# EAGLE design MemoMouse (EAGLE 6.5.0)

## Sheet 1 of 2: CPU
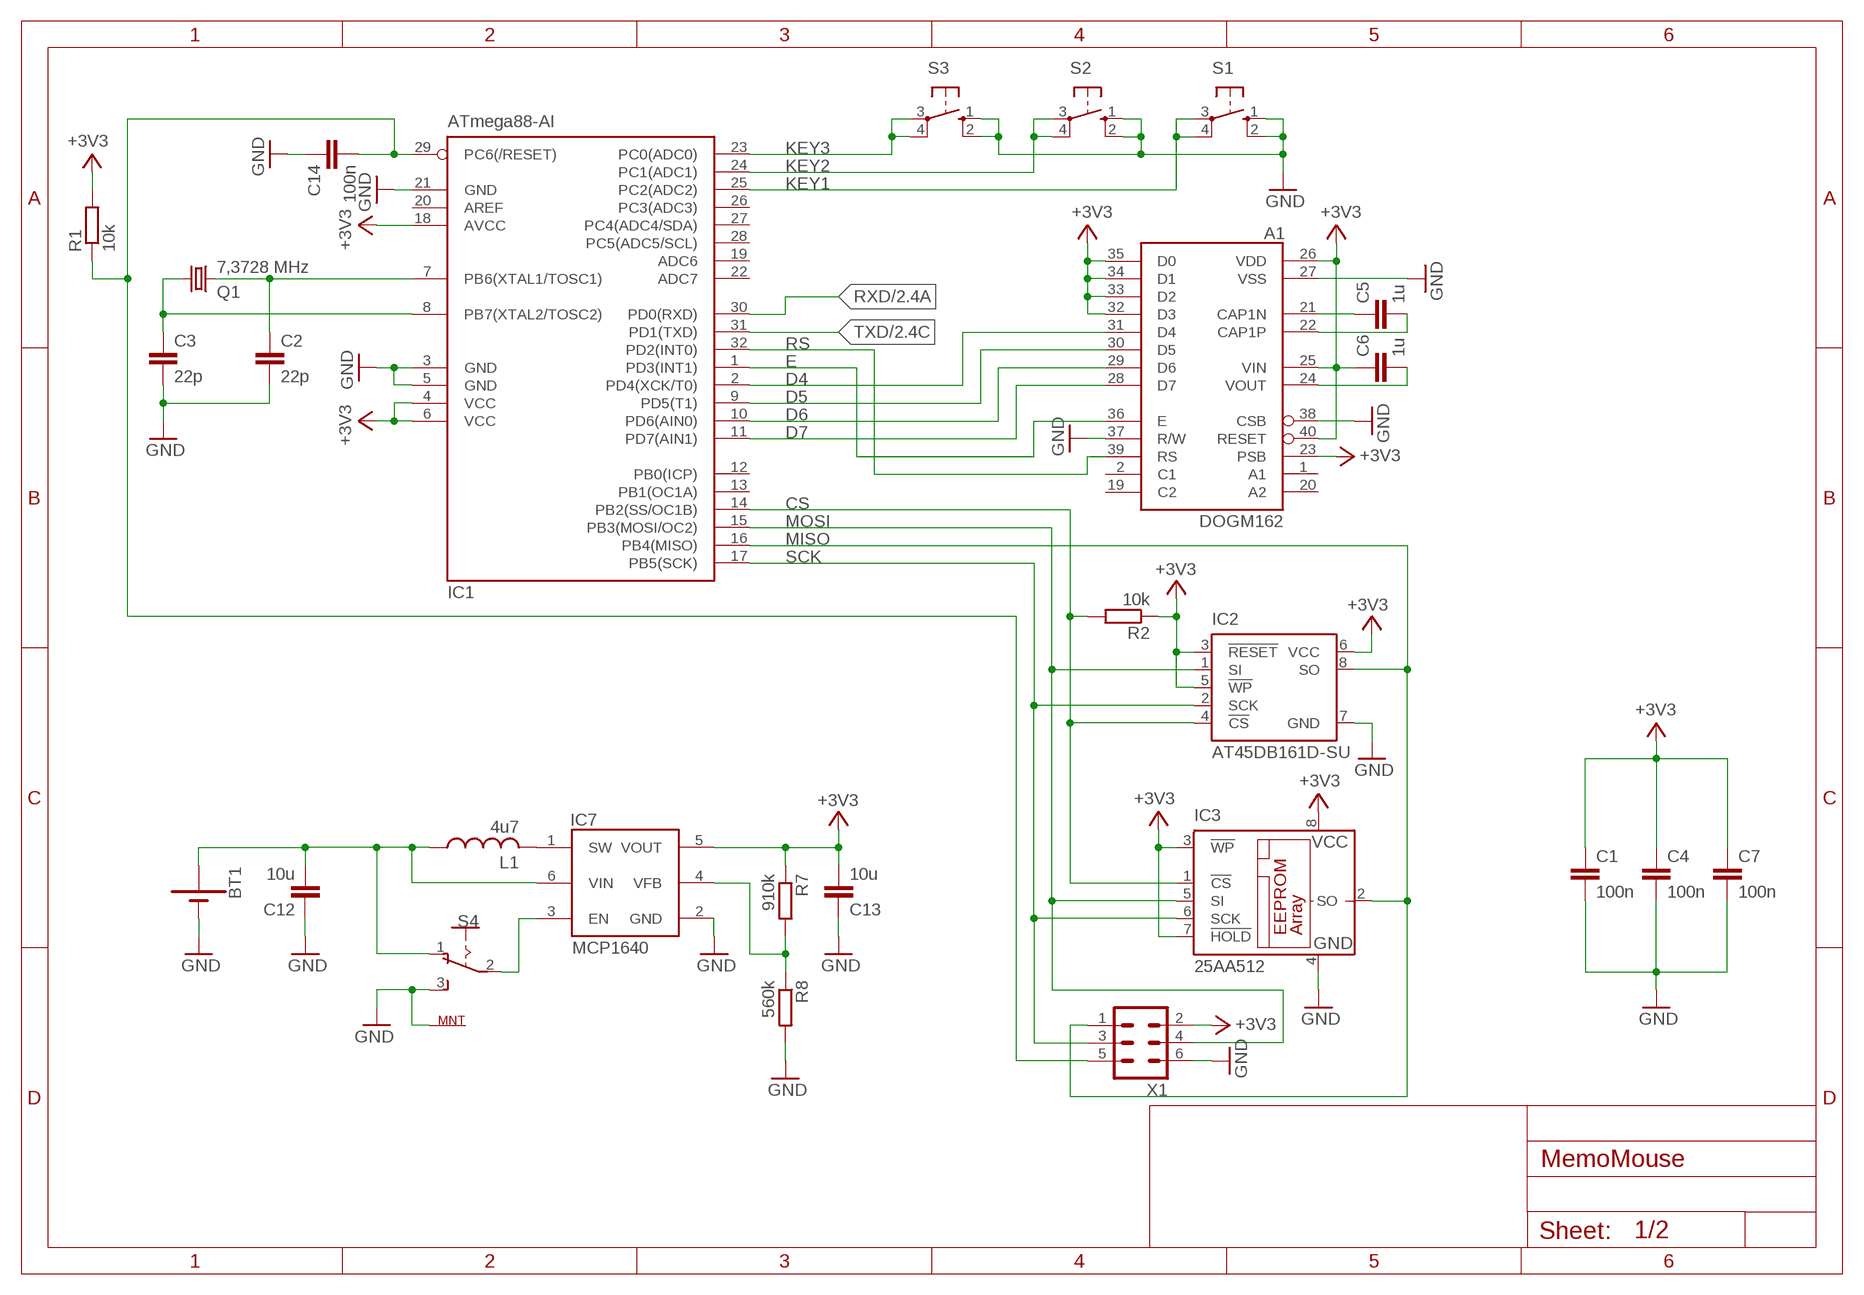
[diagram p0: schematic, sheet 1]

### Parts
A1  DOGM162  SELFMADE_DOGM  [SELFMADE_DOGM]
BT1  BATTERY-AAA_KIT  [BATTERY-AAA-KIT]
C1  100n  C-EUC0603  [C0603]
C2  22p  C-EUC0603  [C0603]
C3  22p  C-EUC0603  [C0603]
C4  100n  C-EUC0603  [C0603]
C5  1u  C-EUC0603  [C0603]
C6  1u  C-EUC0603  [C0603]
C7  100n  C-EUC0603  [C0603]
C12  10u  C-EUC0805K  [C0805K]
C13  10u  C-EUC0805K  [C0805K]
C14  100n  C-EUC0603  [C0603]
IC1  ATmega88-AI  MEGA8-AI  [TQFP32-08]
IC2  AT45DB161D-SU  [8S2]
IC3  25AA512  25AA080SN  [SO-08]
IC7  MCP1640  [SOT23-6]
L1  4u7  L-USL3225M  [L3225M]
Q1  7,3728 MHz  CRYSTALCTS406  [CTS406]
R1  10k  R-EU_R0603  [R0603]
R2  10k  R-EU_R0603  [R0603]
R7  910k  R-EU_R0603  [R0603]
R8  560k  R-EU_R0603  [R0603]
S1  10-XX  [B3F-10XX]
S2  10-XX  [B3F-10XX]
S3  10-XX  [B3F-10XX]
S4  M251SW_H  [MINI_SWITCH]
X1  MICROMATCH06  [MICROMATCH_SMD6]

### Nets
!RESET: C14.2 IC1.29(PC6(/RESET)) R1.1 X1.5
+3V3: A1.23(PSB) A1.25(VIN) A1.26(VDD) A1.32(D3) A1.33(D2) A1.34(D1) A1.35(D0) A1.40(RESET) C1.1 C4.1 C6.1 C7.1 C13.2 IC1.4(VCC) IC1.6(VCC) IC1.18(AVCC) IC2.3(!RESET) IC2.5(!WP) IC2.6(VCC) IC3.3(!WP) IC3.7(!HOLD) IC3.8(VCC) IC7.5(VOUT) R1.2 R2.1 R7.1 X1.2 ; also sheet 2
CS: IC1.14(PB2(SS/OC1B)) IC2.4(!CS) IC3.1(!CS) R2.2
D4: A1.31(D4) IC1.2(PD4(XCK/T0))
D5: A1.30(D5) IC1.9(PD5(T1))
D6: A1.29(D6) IC1.10(PD6(AIN0))
D7: A1.28(D7) IC1.11(PD7(AIN1))
E: A1.36(E) IC1.1(PD3(INT1))
GND: A1.27(VSS) A1.37(R/W) A1.38(CSB) BT1.N1(-) BT1.N2(-) C1.2 C2.2 C3.2 C4.2 C7.2 C12.1 C13.1 C14.1 IC1.3(GND) IC1.5(GND) IC1.21(GND) IC2.7(GND) IC3.4(GND) IC7.2(GND) R8.2 S1.1(S) S1.2(S1) S2.1(S) S2.2(S1) S3.1(S) S3.2(S1) S4.3(S) S4.M1(MNT) S4.M2(MNT) X1.6 ; also sheet 2
KEY1: IC1.25(PC2(ADC2)) S1.3(P) S1.4(P1)
KEY2: IC1.24(PC1(ADC1)) S2.3(P) S2.4(P1)
KEY3: IC1.23(PC0(ADC0)) S3.3(P) S3.4(P1)
MISO: IC1.16(PB4(MISO)) IC2.8(SO) IC3.2(SO) X1.1
MOSI: IC1.15(PB3(MOSI/OC2)) IC2.1(SI) IC3.5(SI) X1.4
N$8: IC7.1(SW) L1.2
N$9: A1.21(CAP1N) C5.1
N$10: A1.22(CAP1P) C5.2
N$11: A1.24(VOUT) C6.2
N$12: C2.1 IC1.7(PB6(XTAL1/TOSC1)) Q1.3
N$13: C3.1 IC1.8(PB7(XTAL2/TOSC2)) Q1.1
N$15: IC7.4(VFB) R7.2 R8.1
N$16: BT1.P1(+) BT1.P2(+) C12.2 IC7.6(VIN) L1.1 S4.1(O)
N$17: IC7.3(EN) S4.2(P)
RS: A1.39(RS) IC1.32(PD2(INT0))
RXD: IC1.30(PD0(RXD)) ; also sheet 2
SCK: IC1.17(PB5(SCK)) IC2.2(SCK) IC3.6(SCK) X1.3
TXD: IC1.31(PD1(TXD)) ; also sheet 2
Unconnected: A1.1(A1) A1.2(C1) A1.19(C2) A1.20(A2) IC1.12(PB0(ICP)) IC1.13(PB1(OC1A)) IC1.19(ADC6) IC1.20(AREF) IC1.22(ADC7) IC1.26(PC3(ADC3)) IC1.27(PC4(ADC4/SDA)) IC1.28(PC5(ADC5/SCL))

## Sheet 2 of 2: IO
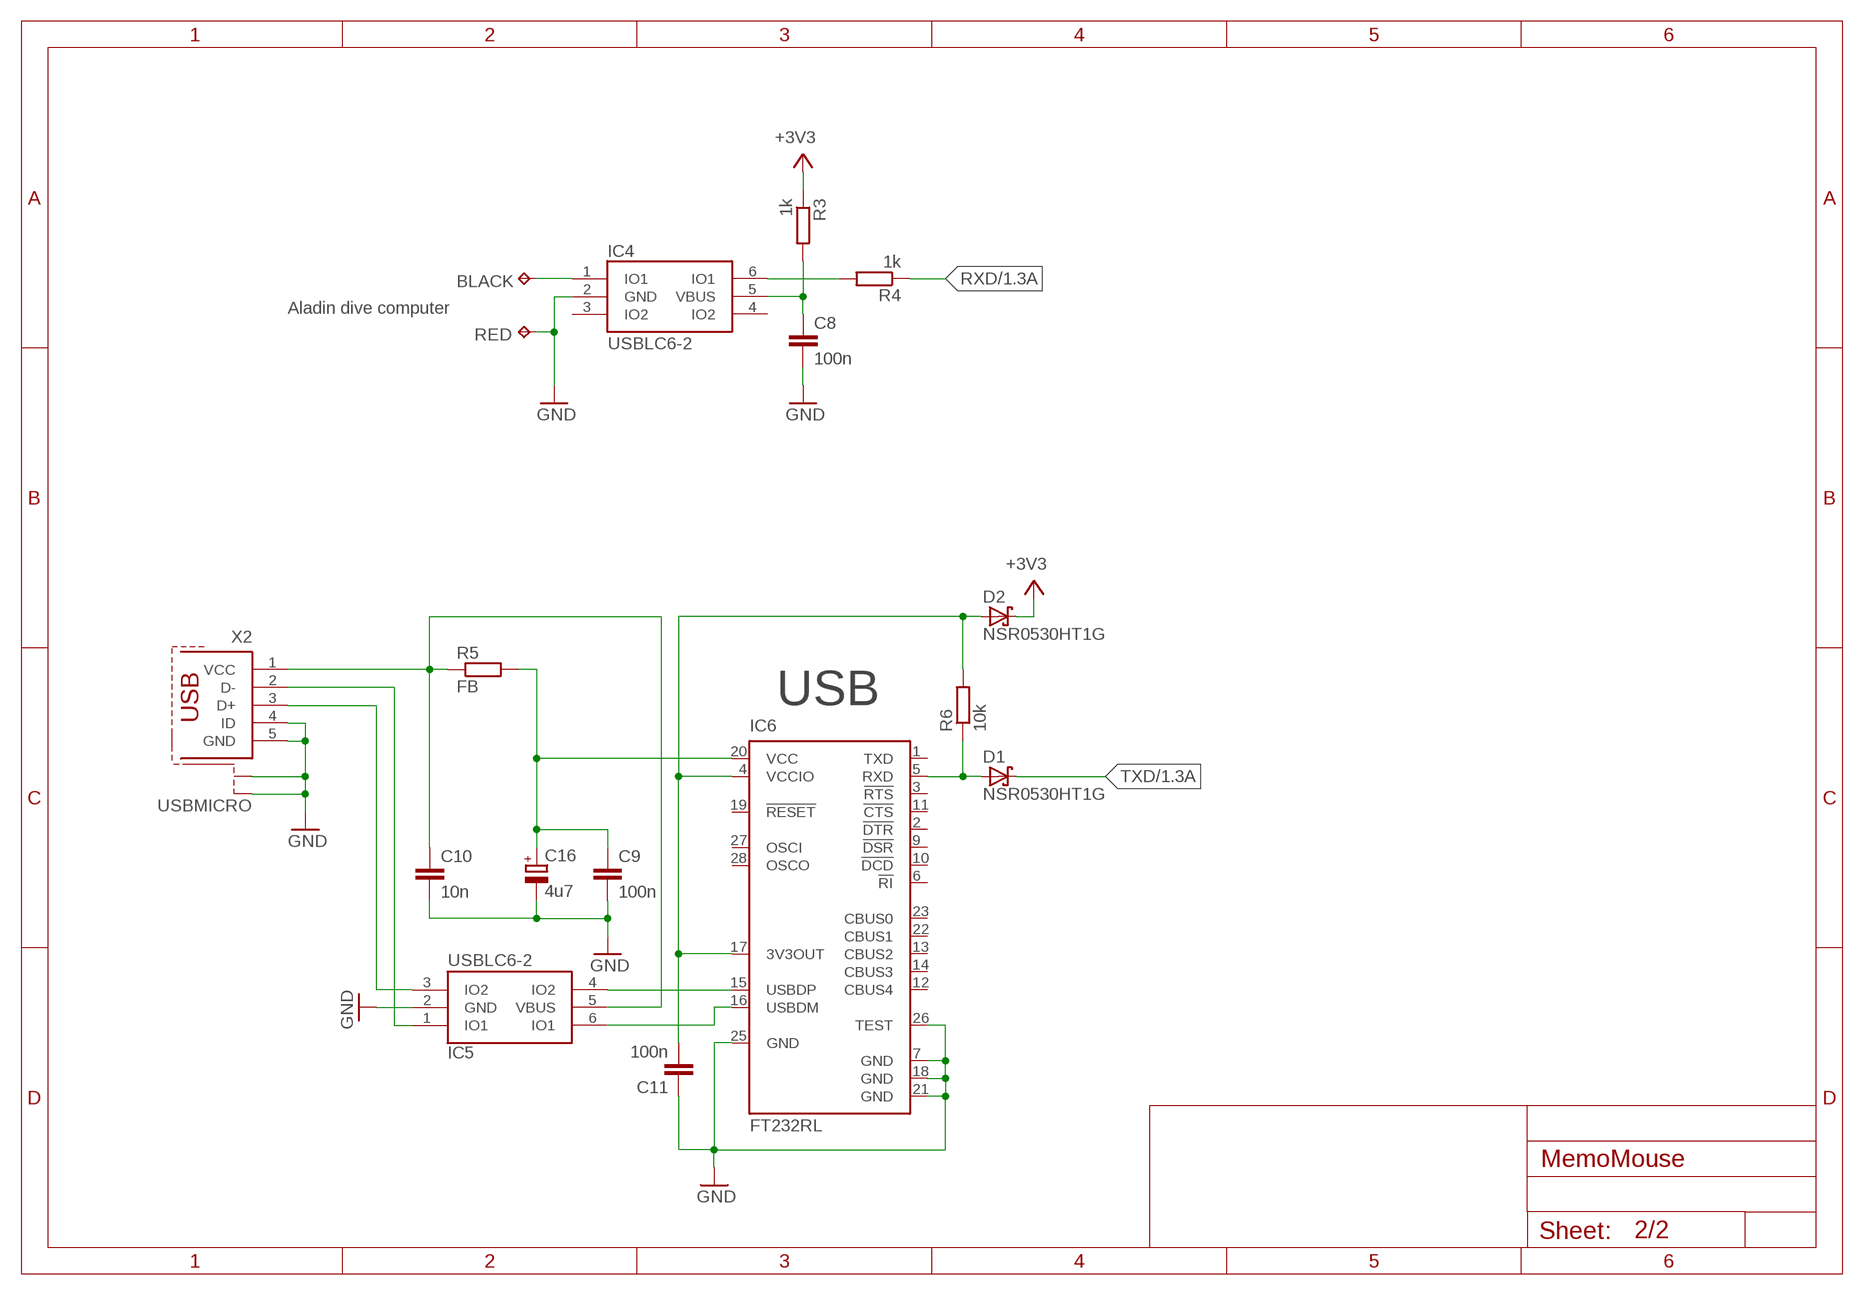
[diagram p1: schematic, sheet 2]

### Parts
BLACK  TPPAD1-13  [P1-13]
C8  100n  C-EUC0603  [C0603]
C9  100n  C-EUC0603  [C0603]
C10  10n  C-EUC0603  [C0603]
C11  100n  C-EUC0603  [C0603]
C16  4u7  CPOL-EUSMCA  [SMC_A]
D1  NSR0530HT1G  DIODE-SCHOTTKYSOD323  [SOD323]
D2  NSR0530HT1G  DIODE-SCHOTTKYSOD323  [SOD323]
IC4  USBLC6-2  [SOT23-6]
IC5  USBLC6-2  [SOT23-6]
IC6  FT232RL  [SSOP28]
R3  1k  R-EU_R0603  [R0603]
R4  1k  R-EU_R0603  [R0603]
R5  FB  R-EU_R0805  [R0805]
R6  10k  R-EU_R0603  [R0603]
RED  TPPAD1-13  [P1-13]
X2  USBMICRO  [MOLEX_USB_MICRO_SD-47346-001]

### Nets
+3V3: D2.C R3.1 ; also sheet 1
GND: C8.2 C9.2 C10.2 C11.1 C16.- IC4.2(GND) IC5.2(GND) IC6.7(GND) IC6.18(GND) IC6.21(GND) IC6.25(GND) IC6.26(TEST) RED.TP X2.4(ID) X2.5(GND) X2.M0(S1) X2.M1(S1) X2.M2(S1) X2.M3(S1) X2.M4(S2) X2.M5(S2) X2.M6(S2) X2.M7(S2) X2.M8(S1) X2.M9(S1) X2.M10(S2) X2.M11(S2) ; also sheet 1
N$1: C8.1 IC4.5(VBUS) R3.2
N$2: IC4.6(IO1) R4.2
N$3: BLACK.TP IC4.1(IO1)
N$4: C10.1 IC5.5(VBUS) R5.1 X2.1(VCC)
N$5: D1.A IC6.5(RXD) R6.1
N$6: IC5.4(IO2) IC6.15(USBDP)
N$7: IC5.6(IO1) IC6.16(USBDM)
N$19: C9.1 C16.+ IC6.20(VCC) R5.2
N$20: IC5.1(IO1) X2.2(D-)
N$37: IC5.3(IO2) X2.3(D+)
N$86: C11.2 D2.A IC6.4(VCCIO) IC6.17(3V3OUT) R6.2
RXD: R4.1 ; also sheet 1
TXD: D1.C ; also sheet 1
Unconnected: IC4.3(IO2) IC4.4(IO2) IC6.1(TXD) IC6.2(!DTR) IC6.3(!RTS) IC6.6(!RI) IC6.9(!DSR) IC6.10(!DCD) IC6.11(!CTS) IC6.12(CBUS4) IC6.13(CBUS2) IC6.14(CBUS3) IC6.19(!RESET) IC6.22(CBUS1) IC6.23(CBUS0) IC6.27(OSCI) IC6.28(OSCO)

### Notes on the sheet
- Aladin dive computer
- USB

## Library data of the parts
A1 = brunner:SELFMADE_DOGM
BLACK RED = testpad:TP: Test pad
BT1 = SparkFun-Batteries:BATTERY: Battery - Single Cell; PROD_ID: BATT-08571; SF_SKU: PRT-12718
C1-C14 = rcl:C-EU: CAPACITOR, European symbol
C16 = rcl:CPOL-EU: POLARIZED CAPACITOR, European symbol; OC_FARNELL: unknown
D1 D2 = brunner:DIODE-SCHOTTKY
IC1 = atmel:MEGA8: MICROCONTROLLER 8 Kbytes FLASH, 1 kbytes SRAM, 512 bytes EEPROM, USART, 6-channel 10 bit ADC, 2-channel 8 bit ADC Pin compatible with Atmega48, ATMega88, ATMega168 Source: avr.lbr; MPN: ATMEGA8-16AU; OC_FARNELL: 9171371; OC_NEWARK: 73M8863
IC2 = atmel:AT45DB161D: 16-megabit 2.5V or 2.7V DataFlash Source: http://www.atmel.com/dyn/resources/prod_documents/doc3500.pdf; MF: ATMEL; MPN: AT45DB161D-SU; OC_FARNELL: 1455040
IC3 = microchip:25*: Serial EEPROM 4K/ 8K , SPI bus; MF: MICROCHIP; MPN: 25AA080/SN; OC_FARNELL: 1816072; OC_NEWARK: 92C7351
IC4 IC5 = Brunner_KMT:USBLC6-2
IC6 = ftdichip:FT232R: Source: http://www.ftdichip.com/Documents/DataSheets/DS_FT232R_v104.pdf; MF: FTDI; MPN: FT232RL; OC_FARNELL: 1146032; OC_NEWARK: 91K9918
IC7 = brunner:MCP1640
L1 = rcl:L-US: INDUCTOR, American symbol
Q1 = crystal:CRYSTAL: CRYSTAL; OC_FARNELL: unknown; OC_NEWARK: unknown
R1-R8 = rcl:R-EU_: RESISTOR, European symbol
S1-S3 = switch-omron:10-XX: OMRON SWITCH; MPN: B3F-1000; OC_FARNELL: 176432; OC_NEWARK: 36M3542
S4 = brunner:M251: SLIDING SWITCH Mors, distributor Buerklin, 11G702
X1 = brunner:MICROMATCH06
X2 = brunner:USB

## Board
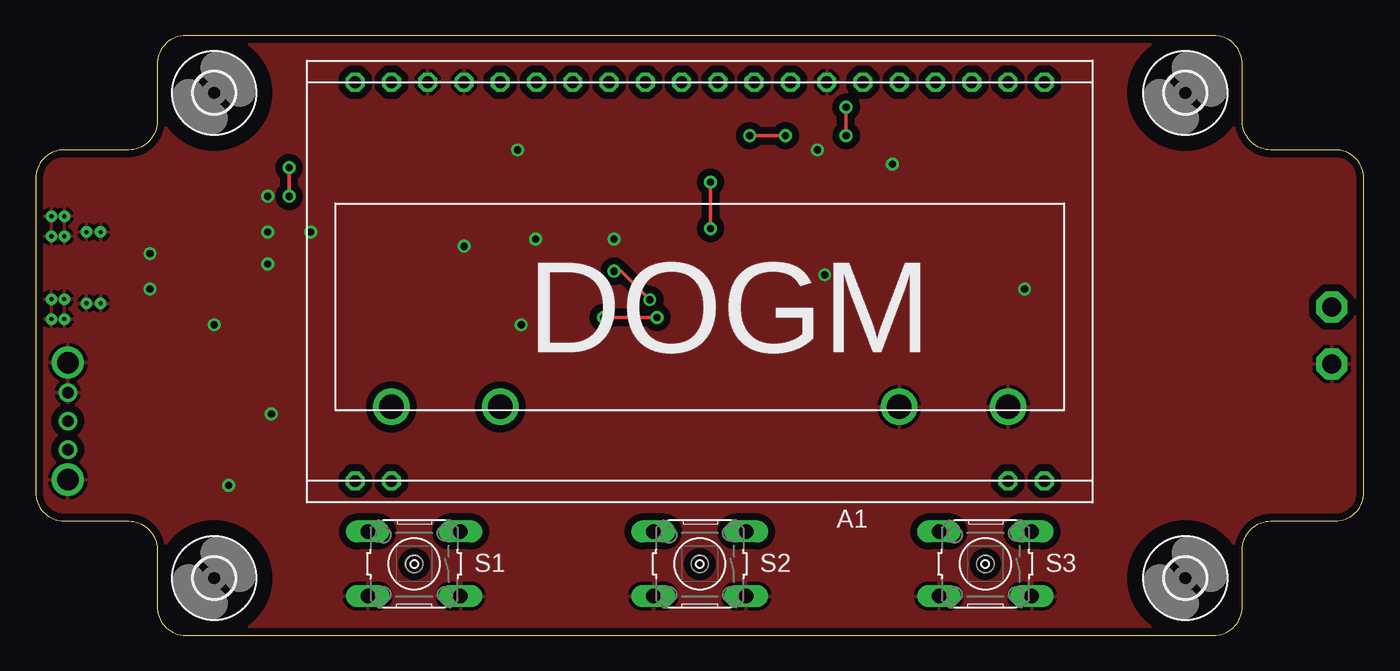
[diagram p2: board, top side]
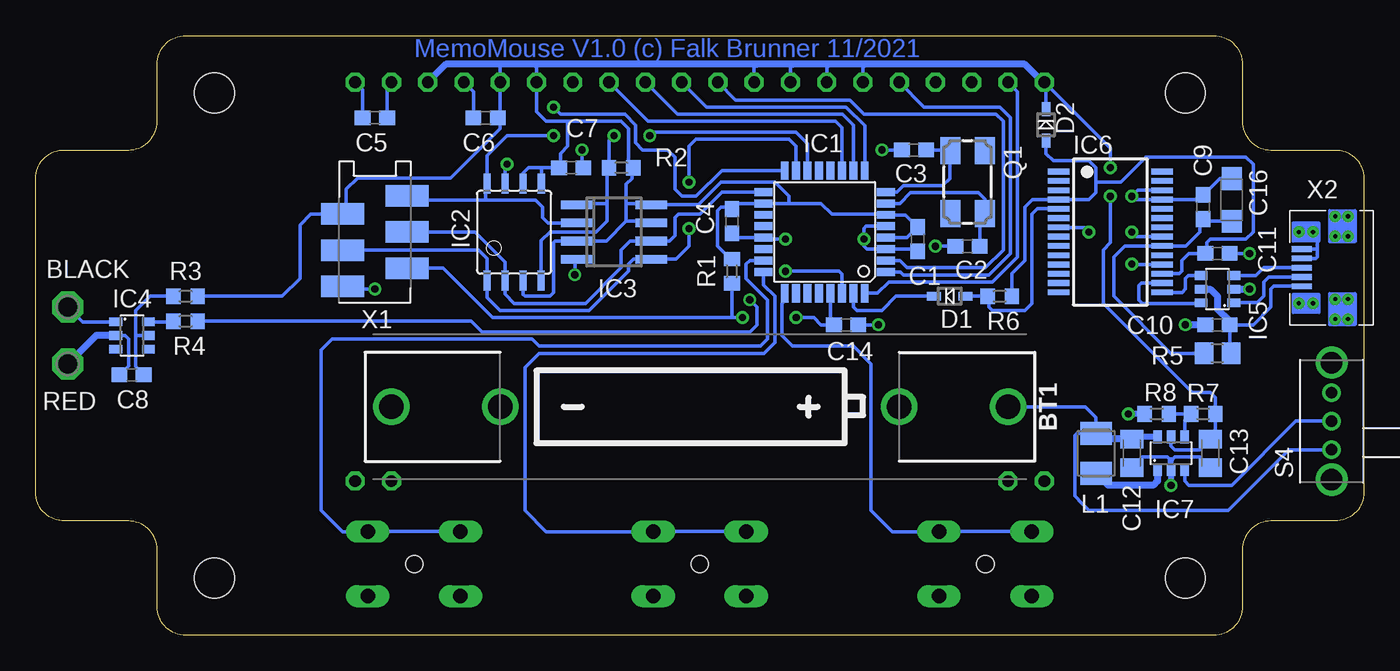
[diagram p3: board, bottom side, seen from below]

Size 93 x 42 mm. Coordinates in mm from the lower left corner, seen from the top.
Outline: 10.5,0 82.5,0 arc90 84.5,2 84.5,6 arc-90 86.5,8 91,8 arc90 93,10 93,32 arc90 91,34 86.5,34 arc-90 84.5,36 84.5,40 arc90 82.5,42 10.5,42 arc90 8.5,40 8.5,36 arc-90 6.5,34 2,34 arc90 0,32 0,10 arc90 2,8 6.5,8 arc-90 8.5,6 8.5,2 arc90 10.5,0
Copper layers (1*16): Top 0.035mm / dielectric 1.5mm / Bottom 0.035mm
Design rules "default *": minimum track width 0.25mm, minimum drill 0.5mm, track to track 0.25mm, track to pad 0.25mm, pad to pad 0.23mm, via to via 0.25mm, smd to smd 0.2mm, copper to edge 0.5mm, drill to drill 8mil, minimum pad ring 10mil, minimum via ring 8mil, stop-mask expansion 4mil, vias tented up to drill 0mil, thermal gap 10mil
Holes 1.2 mm at 26.5,5 46.5,5 66.5,5

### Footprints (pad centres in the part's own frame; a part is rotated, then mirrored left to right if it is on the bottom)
SELFMADE_DOGM = drill 0.813 octagon: 1 -24.13,-12.2; 2 -21.59,-12.2; 19 21.59,-12.2; 20 24.13,-12.2; 21 24.13,15.74; 22 21.59,15.74; 23 19.05,15.74; 24 16.51,15.74; 25 13.97,15.74; 26 11.43,15.74; 27 8.89,15.74; 28 6.35,15.74; 29 3.81,15.74; 30 1.27,15.74; 31 -1.27,15.74; 32 -3.81,15.74; 33 -6.35,15.74; 34 -8.89,15.74; 35 -11.43,15.74; 36 -13.97,15.74; 37 -16.51,15.74; 38 -19.05,15.74; 39 -21.59,15.74; 40 -24.13,15.74
P1-13 = drill 1.321 pad 2.159 octagon: TP 0,0
BATTERY-AAA-KIT = drill 1.702: N1 13.97,0; N2 21.59,0; P1 -21.59,0; P2 -13.97,0
C0603 = smd 1.1 x 1: 1 -0.85,0; 2 0.85,0
C0805K = smd 1.3 x 1.6: 1 -1,0; 2 1,0
SMC_A = smd 1.6 x 1.4: + -1.5,0; - 1.5,0
SOD323 = smd 1 x 0.6: A 1.1,0; C -1.1,0
TQFP32-08 = smd 1.27 x 0.559: 1 -4.293,2.8; 2 -4.293,2; 3 -4.293,1.2; 4 -4.293,0.4; 5 -4.293,-0.4; 6 -4.293,-1.2; 7 -4.293,-2; 8 -4.293,-2.8; 17 4.293,-2.8; 18 4.293,-2; 19 4.293,-1.2; 20 4.293,-0.4; 21 4.293,0.4; 22 4.293,1.2; 23 4.293,2; 24 4.293,2.8 | smd 0.559 x 1.27: 9 -2.8,-4.293; 10 -2,-4.293; 11 -1.2,-4.293; 12 -0.4,-4.293; 13 0.4,-4.293; 14 1.2,-4.293; 15 2,-4.293; 16 2.8,-4.293; 25 2.8,4.293; 26 2,4.293; 27 1.2,4.293; 28 0.4,4.293; 29 -0.4,4.293; 30 -1.2,4.293; 31 -2,4.293; 32 -2.8,4.293
8S2 = smd 0.5 x 1.4: 1 -1.905,-3.404; 2 -0.645,-3.404; 3 0.625,-3.404; 4 1.895,-3.404; 5 1.905,3.404; 6 0.635,3.404; 7 -0.635,3.404; 8 -1.905,3.404
SO-08 = smd 0.6 x 2.2: 1 -1.905,-2.6; 2 -0.635,-2.6; 3 0.635,-2.6; 4 1.905,-2.6; 5 1.905,2.6; 6 0.635,2.6; 7 -0.635,2.6; 8 -1.905,2.6
SOT23-6 = smd 0.6 x 0.9: 1 -0.95,-1.15; 2 0,-1.15; 3 0.95,-1.15; 4 0.95,1.15; 5 0,1.15; 6 -0.95,1.15
SSOP28 = smd 0.4 x 1.5: 1 -4.225,-3.625; 2 -3.575,-3.625; 3 -2.925,-3.625; 4 -2.275,-3.625; 5 -1.625,-3.625; 6 -0.975,-3.625; 7 -0.325,-3.625; 8 0.325,-3.625; 9 0.975,-3.625; 10 1.625,-3.625; 11 2.275,-3.625; 12 2.925,-3.625; 13 3.575,-3.625; 14 4.225,-3.625; 15 4.225,3.625; 16 3.575,3.625; 17 2.925,3.625; 18 2.275,3.625; 19 1.625,3.625; 20 0.975,3.625; 21 0.325,3.625; 22 -0.325,3.625; 23 -0.975,3.625; 24 -1.625,3.625; 25 -2.275,3.625; 26 -2.925,3.625; 27 -3.575,3.625; 28 -4.225,3.625
L3225M = smd 1.6 x 2.2: 1 -1.4,0; 2 1.4,0
CTS406 = smd 1.9 x 1.4: 1 -2.2,-1.2; 2 2.2,-1.2; 3 2.2,1.2; 4 -2.2,1.2
R0603 = smd 1 x 1.1: 1 -0.85,0; 2 0.85,0
R0805 = smd 1.3 x 1.5: 1 -0.95,0; 2 0.95,0
B3F-10XX = drill 1.016 long: 1 -3.251,2.261; 2 3.251,2.261; 3 -3.251,-2.261; 4 3.251,-2.261
MINI_SWITCH = drill 0.8: 1 -2,0; 2 0,0; 3 2,0 | drill 1.5: M1 -4.1,0; M2 4.1,0
2,8 = hole 2.8: 0,0
MICROMATCH_SMD6 = smd 1.5 x 3: 1 2.54,-2.25; 2 1.27,2.25; 3 0,-2.25; 4 -1.27,2.25; 5 -2.54,-2.25; 6 -3.81,2.25
MOLEX_USB_MICRO_SD-47346-001 = smd 0.4 x 1.4: 1 -1.3,2.85; 2 -0.65,2.85; 3 0,2.85; 4 0.65,2.85; 5 1.3,2.85 | drill 0.3: M0 -3.6,0.5; M1 -2.2,0.5; M2 -3.6,-0.4; M3 -2.2,-0.4; M4 2.2,0.5; M5 3.6,0.5; M6 2.2,-0.4; M7 3.6,-0.4; M8 -2.5,3.05; M9 -2.5,2.05; M10 2.5,3.05; M11 2.5,2.05

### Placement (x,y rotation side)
A1  46.5,23 0 top
BLACK  90.75,23 0 bottom
BT1  46.5,16 180 bottom
C1  31.25,27.75 270 bottom
C2  27.75,27.25 180 bottom
C3  31.5,34 180 bottom
C4  44.25,29 270 bottom
C5  69.25,36.25 0 bottom
C6  61.5,36.25 180 bottom
C7  55.5,32.75 0 bottom
C8  86.28,18.25 180 bottom
C9  11.25,30 90 bottom
C10  10.25,21.75 180 bottom
C11  10.25,26.75 180 bottom
C12  16.25,12.75 90 bottom
C13  10.75,12.75 90 bottom
C14  36.25,21.75 180 bottom
C16  9.25,30.5 90 bottom
D1  29,23.75 0 bottom
D2  22.25,35.75 270 bottom
IC1  37.75,28.25 180 bottom
IC2  59.5,28.25 0 bottom
IC3  52.5,28.25 270 bottom
IC4  86.25,21 270 bottom
IC5  10.25,24.25 90 bottom
IC6  17.75,28.25 270 bottom
IC7  13.5,12.75 0 bottom
L1  18.75,12.75 270 bottom
Q1  27.75,31.75 270 bottom
R1  44.25,25.5 90 bottom
R2  52,32.75 180 bottom
R3  82.5,23.75 180 bottom
R4  82.5,22 180 bottom
R5  10.25,19.75 180 bottom
R6  25.5,23.75 0 bottom
R7  11.25,15.5 180 bottom
R8  14.5,15.5 180 bottom
RED  90.75,19 0 bottom
S1  26.5,5 180 top
S2  46.5,5 180 top
S3  66.5,5 180 top
S4  2.25,15 90 bottom
U$1  [2,8]  12.5,4 0 top
U$2  [2,8]  12.5,38 0 top
U$3  [2,8]  80.5,38 0 top
U$4  [2,8]  80.5,4 0 top
U$5  [A5L-LOC]  not placed on the board
U$6  [A5L-LOC]  not placed on the board
X1  69.25,28.25 90 bottom
X2  1.5,25.75 90 bottom

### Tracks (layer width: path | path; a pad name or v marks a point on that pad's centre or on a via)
!RESET  (via drill 0.5)
  Top 0.25: v43.5,22.25 v39.75,22.25
  Bottom 0.25: R1.1 44.25,22.25 | v43.5,22.25 44.25,22.25 | IC1.29 37.35,22 C14.2 38,21.75 38.5,22.25 v39.75,22.25 | 44.25,22.25 61,22.25 64.46,25.71 X1.5
+3V3  (via drill 0.5)
  Top 0.25: v17.75,30.75 v17.75,32.75
  Bottom 0.25: A1.40 22.49,38.74 | 60.5,40 60.47,39.97 A1.25 60.47,36.43 C6.1 60.5,36.1 60.5,35.5 63.96,32.04 70.46,32.04 71.25,31.25 71.25,29.77 X1.2 73.73,29.52 74.5,28.75 74.5,25 75.75,23.75 R3.1 | 58,40 57.93,39.93 A1.26 57.93,36.68 57.25,36 55.75,36 | A1.35 35.07,39.93 35,40 | A1.34 37.61,39.89 37.5,40 | A1.33 40.15,39.85 40,40 | A1.32 42.69,39.81 42.5,40 | 55.75,36 52,36 51.5,35.5 51.5,33 51.25,32.75 R2.1 51.25,32.65 51.25,32 51.65,31.6 51.65,30.25 | 51.65,30.25 51.65,29 | 40.25,30.25 38,30.25 37.25,29.5 34,29.5 33.95,29.45 IC1.6 32.1,29.45 C1.1 32,27.85 IC1.4 | 40.25,30.25 IC1.18 43.85,30.25 C4.1 44.4,30 45,30 45.25,29.75 45.25,27.25 44.35,26.35 R1.2 | 40.25,30.25 40.25,30.75 41.25,31.75 45,31.75 46.59,30.16 IC3.8 49.84,30.16 49.75,30.25 51.65,30.25 | IC2.3 58.88,23.88 58.75,23.75 57,23.75 56.75,24 56.75,27.5 56.63,27.61 IC3.3 53.03,27.61 51.65,29 | 55.75,36 55.75,34.25 56.25,33.75 56.25,32.85 C7.1 57.5,32.75 | R7.1 10.4,16.65 10.75,17 12,17 18.25,23.25 18.25,27 17.75,27.5 v17.75,30.75 | IC7.5 13.5,13.25 13.25,13 11.5,13 C13.2 | D2.C 22.25,38.62 A1.40 | A1.40 | IC3.7 50.38,28.89 50.5,29 51.65,29 | 57.5,32.75 58.5,32.75 58.87,32.38 IC2.6 | IC2.5 57.59,32.66 57.5,32.75 | v17.75,32.75 17.75,34.12 A1.40
  Bottom 0.256: R7.1 10.4,14.1 C13.2
  Bottom 0.5: 22.49,38.74 23.75,40 35,40 37.5,40 40,40 42.5,40 58,40 60.5,40 64.29,40 A1.23
CS  (via drill 0.5)
  Top 0.25: v50,35 v52.5,35
  Bottom 0.25: IC1.14 38.95,34.45 39.75,35.25 49.75,35.25 v50,35 | v52.5,35 52.85,34.65 R2.2 53,32.6 53,30.25 | IC2.4 57.6,27.64 57,28.25 53.75,28.25 53,29 53,30.25 | IC3.1 54.84,30.16 54.75,30.25 53,30.25
D4
  Bottom 0.25: IC1.2 32.5,26.25 32,25.75 26.5,25.75 25.25,27 25.25,36 25.75,36.5 35,36.5 36,37.5 43.99,37.5 A1.31
D5
  Bottom 0.25: IC1.9 34.95,35.7 36.25,37 46.03,37 A1.30
D6
  Bottom 0.25: IC1.10 35.75,35.75 36.5,36.5 48.07,36.5 A1.29
D7
  Bottom 0.25: IC1.11 36.55,35.55 37,36 50.11,36 A1.28
E
  Bottom 0.25: IC1.1 32.45,25.45 32.25,25.25 26.25,25.25 24.75,26.75 24.75,36.25 25.5,37 30.79,37 A1.36
GND  (via drill 0.5)
  Bottom 0.25: IC1.5 34.85,28.65 35,28.5 v35,27.75 35,27.25 34.8,27.05 IC1.3 31.4,27.05 C1.2 | C4.2 43.95,27.85 IC1.21 41.6,27.85 41.5,27.75 v40.5,27.75 | C7.2 54.65,32.9 54.75,33 v54.75,34 | IC6.7 19.57,28.57 v19.25,28.25 | X2.4 3.35,26.4 3.25,26.5 3.25,27 | 3.25,27 3.25,27.95 X2.M11 | X2.5 3.3,27.05 3.25,27 | IC6.18 16.23,25.98 v16.25,26 | IC6.21 15.93,27.93 v16.25,28.25 | C14.1 v34,21.75 | C2.2 v30,27.25 | IC6.26 15.82,31.18 v16.25,30.75 16.02,30.52 IC6.25 11.72,30.52 11.5,30.75 11.35,30.75 C9.2 10.1,32 C16.- | IC4.2 86.75,21 86.5,20.75 86.5,18.88 C8.2 | C11.1 v8,26.75 | C12.1 15.5,12.5 13.75,12.5 13.5,12.25 13.25,12.5 11.5,12.5 C13.1 | X1.6 71.44,24.44 71.25,24.25 v69.25,24.25 | v55.25,25.25 55.25,26.2 IC3.4 | IC2.7 60.13,32.87 v60,33 | C3.2 v33.75,34
  Bottom 0.406: v13.5,10.5 IC7.2 13.5,12.25 | R8.2 v16.5,15.5
  Bottom 0.5: C10.2 v12.5,21.75 | IC5.2 v8,24.25 | IC4.2 88.75,21 RED.TP
  pour Top (isolate 0.5): 0,42 93,42 93,0 0,0
KEY1
  Bottom 0.25: S1.4 S1.3 29.76,7.25 33,7.25 34.5,8.75 34.5,19 35.75,20.25 40,20.25 40.75,21 40.75,23.25 40.55,23.45 IC1.25
KEY2
  Bottom 0.25: S2.4 S2.3 49.76,7.25 57.25,7.25 58.75,8.75 58.75,18.75 57.75,19.75 42,19.75 41.25,20.5 41.25,23.75 42.04,24.54 IC1.24
KEY3
  Bottom 0.25: IC1.23 43,26.25 43.25,26 43.25,25 41.75,23.5 41.75,20.75 42.25,20.25 57.75,20.25 58.25,20.75 72.25,20.75 73,20 73,8.75 71.5,7.25 69.76,7.25 S3.3 S3.4 63.24,7.25
MISO  (via drill 0.5)
  Top 0.25: v56.75,35 v56.75,37
  Bottom 0.25: IC1.16 44.96,32.54 46.75,30.75 47.75,30.75 48.25,31.25 48.25,33.5 48.75,34 50.5,34 51,34.5 51,35.75 51.75,36.5 56.25,36.5 v56.75,37 | v56.75,35 60,35 61.41,33.59 IC2.8 61.41,32.09 61.5,32 61.5,30.5 | 61.5,30.5 66.5,30.5 66.75,30.75 66.96,30.75 X1.1 | 61.5,30.5 58,30.5 57.5,30 57.5,29.25 57.13,28.89 IC3.2
MOSI  (via drill 0.5)
  Top 0.25: v47.25,31.75 v47.25,28.5
  Bottom 0.25: IC1.15 39.75,34.25 40.25,34.75 46.75,34.75 47.25,34.25 v47.25,31.75 | v47.25,28.5 47.25,27.25 48.16,26.34 IC3.5 51.16,26.34 51.5,26 51.5,25.5 54.25,22.75 60.5,22.75 61.41,23.66 IC2.1 61.41,26.41 62,27 70.5,27 70.52,26.98 X1.4
N$1
  Bottom 0.25: IC4.5 86,21 | 86,21 86,18.82 C8.1 | 86,21 86,22.75 85,23.75 R3.2
N$2
  Bottom 0.25: IC4.6 83.4,21.95 R4.2
N$3
  Bottom 0.25: IC4.1 89.7,21.95 BLACK.TP
N$4
  Bottom 0.25: X2.1 6.3,24.45 6.5,24.25 6.5,23 7.75,21.75 C10.1 9.4,19.85 R5.1
  Bottom 0.5: IC5.5 10.75,24.25 10.25,23.75 10.25,22.85 9.4,22 C10.1
N$5
  Bottom 0.25: IC6.5 22.88,29.88 23.25,29.5 23.25,23.25 23.75,22.75 26,22.75 26.25,23 26.25,23.65 R6.1 D1.A
N$6
  Bottom 0.25: IC6.15 12.72,24.02 12.5,24.25 12.5,25 12.3,25.2 IC5.4
N$7
  Bottom 0.25: IC6.16 15.57,24.68 15.75,24.5 15.75,23.5 15.5,23.25 11.45,23.25 IC5.6
N$8
  Bottom 0.5: IC7.1 14.45,10.8 14.75,10.5 17.9,10.5 L1.2
N$9
  Bottom 0.25: C5.1 70.1,38.21 A1.21
N$10
  Bottom 0.25: C5.2 68.4,38.43 A1.22
N$11
  Bottom 0.25: C6.2 62.35,38.08 A1.24
N$12
  Bottom 0.25: IC1.7 32.5,30.25 31.75,31 27,31 26.55,30.55 Q1.3 26.9,29.2 C2.1
N$13
  Bottom 0.25: IC1.8 32.7,31.05 32.25,31.5 29.5,31.5 29,32 29,33.9 Q1.1 29,34 C3.1
N$15
  Bottom 0.256: R8.1 R7.2 12.55,15.05 IC7.4
N$16
  Bottom 0.25: 20.25,9.75 20.25,14 20.1,14.15 L1.1 18.75,15.25 19.5,16 BT1.P1 | S4.1 5.25,13 9.5,8.75 19.25,8.75 19.75,9.25
  Bottom 0.256: 20.25,9.75 19.75,9.25
  Bottom 0.406: IC7.6 16.1,13.9 C12.2
  Bottom 0.5: C12.2 18.35,13.75 L1.1
N$17
  Bottom 0.25: IC7.3 12.55,10.8 12.25,10.5 9.25,10.5 4.75,15 S4.2
N$19
  Bottom 0.25: C16.+ 11.1,29 C9.1 11.5,28.9 11.5,28.25 12.47,27.27 IC6.20 16.73,27.27 17.5,26.5 17.5,23.75 13.5,19.75 R5.2
N$20
  Bottom 0.25: X2.2 6.65,25.1 7,24.75 7,23.75 7.45,23.3 IC5.1
N$37
  Bottom 0.25: X2.3 7,25.75 7.55,25.2 IC5.3
N$86
  Bottom 0.25: IC6.17 12.93,25.32 12.75,25.5 12.75,26.25 12.25,26.75 C11.2 11,26.85 11,27.5 10.75,27.75 8.25,27.75 7.75,28.25 7.75,33 8.25,33.5 15.25,33.5 17,31.75 18.75,31.75 | D2.A 22.25,33.75 21.75,33.25 19.25,33.25 18.75,32.75 18.75,31.75 | 18.75,31.75 18.75,31.02 19.25,30.52 IC6.4 23.23,30.52 23.75,30 23.75,26.25 24.65,25.35 R6.2
RS
  Bottom 0.25: A1.39 24.25,38.08 24.25,26.5 26,24.75 33.25,24.75 34.04,23.96 IC1.32
RXD  (via drill 0.5)
  Top 0.25: v40.5,25.5 41,25.5 v43,23.5
  Bottom 0.25: v43,23.5 42.5,23 42.5,21.75 43,21.25 61.75,21.25 62.5,22 R4.1 | IC1.30 36.55,25.3 36.75,25.5 v40.5,25.5
SCK
  Bottom 0.25: IC1.17 44.95,31.05 46.5,29.5 48,29.5 48.25,29.25 48.25,28 48.63,27.61 IC3.6 51.38,27.61 52,27 52,25.75 54.5,23.25 59.5,23.25 60.15,23.89 IC2.2 60.15,26.14 62.25,28.25 X1.3
TXD
  Bottom 0.25: IC1.31 35.75,23 35.5,22.75 33.75,22.75 32.75,23.75 D1.C

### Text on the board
Bottom: MemoMouse V1.0 (c) Falk Brunner 11/2021
bStop: MemoMouse V1.0 (c) Falk Brunner 11/2021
